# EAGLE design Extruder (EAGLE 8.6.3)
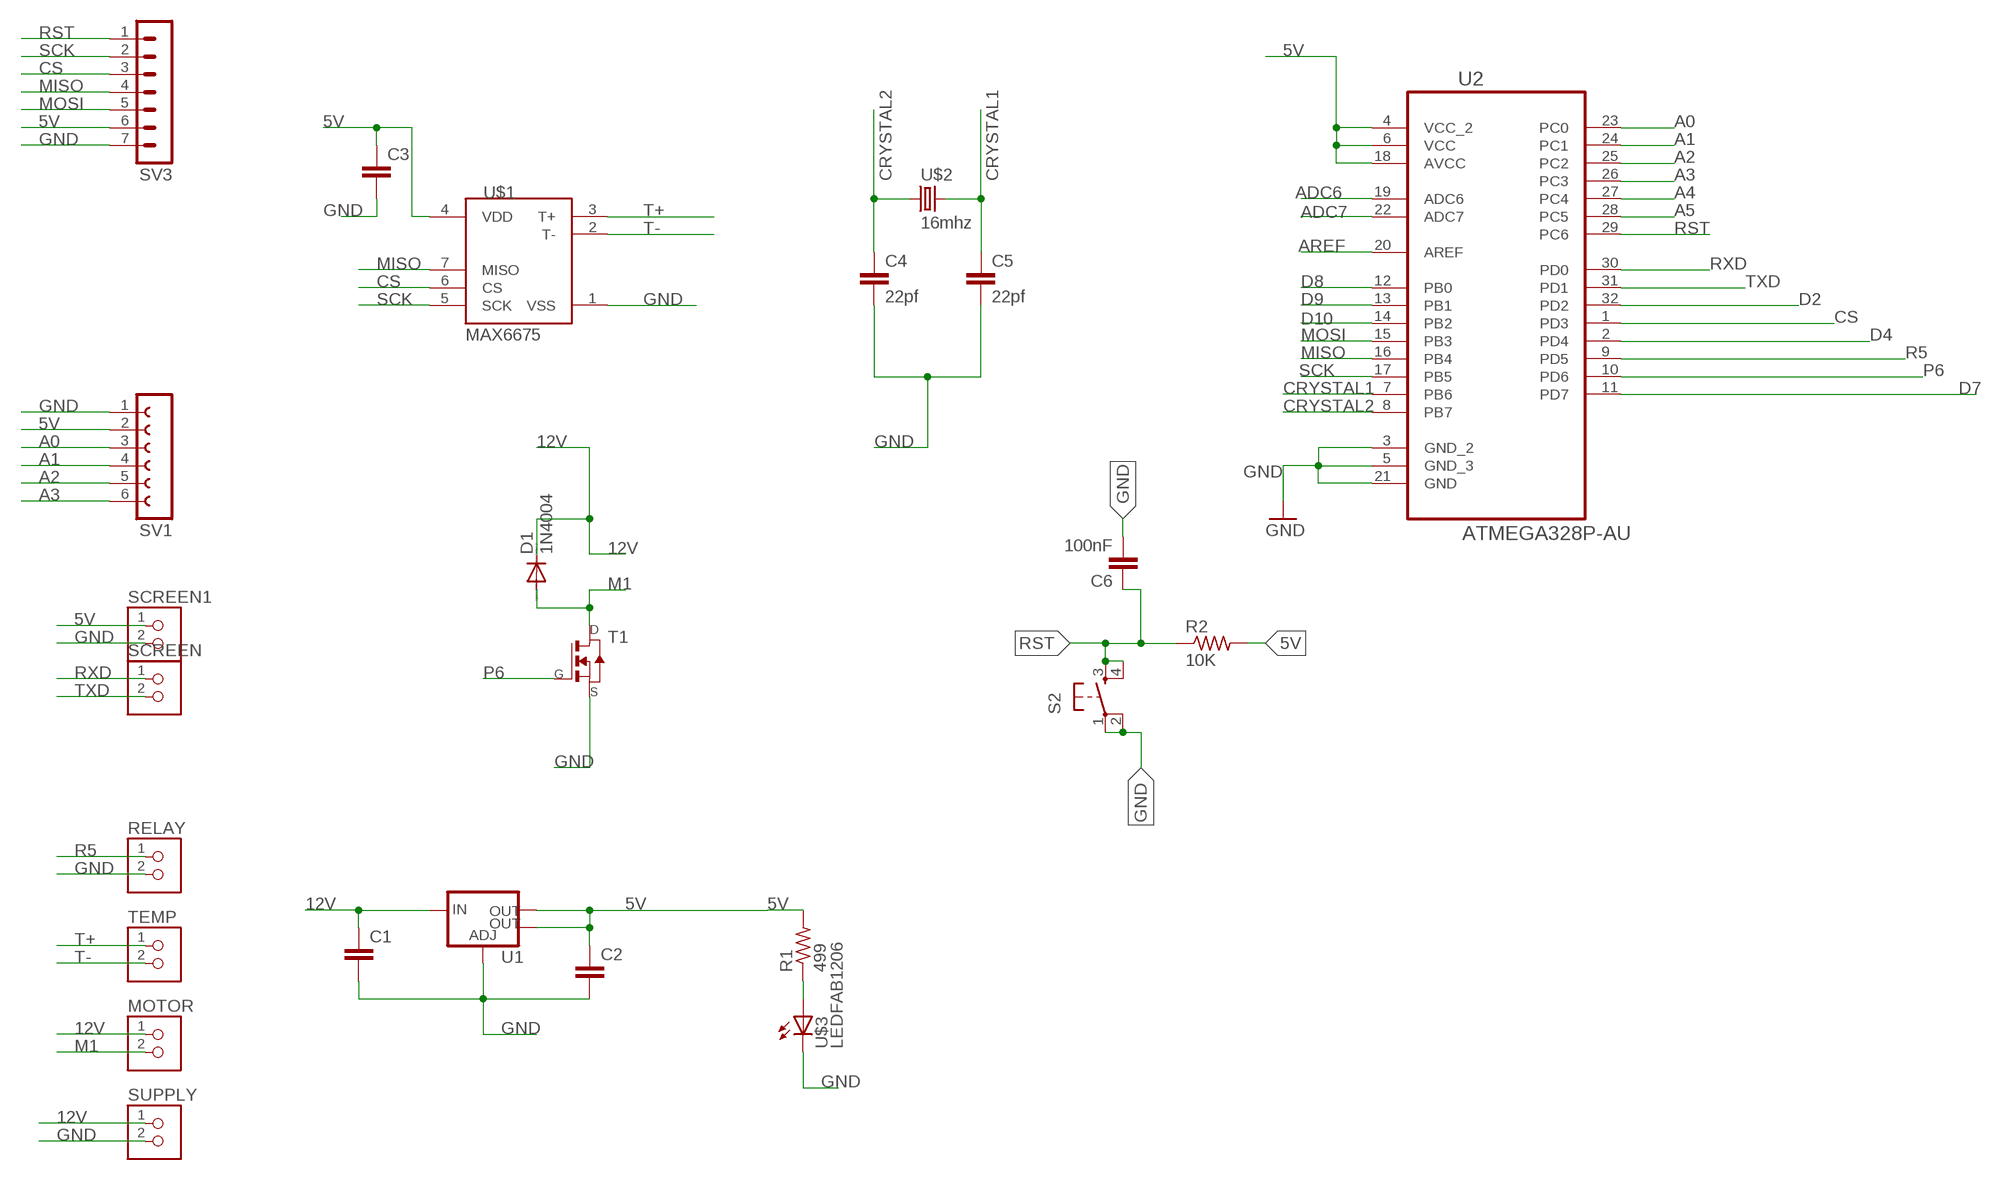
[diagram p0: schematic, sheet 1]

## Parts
C1  C-EUC1206  [C1206]
C2  C-EUC1206  [C1206]
C3  C-EUC1206  [C1206]
C4  22pf  C-EUC1206  [C1206]
C5  22pf  C-EUC1206  [C1206]
C6  100nF  CAP1206  [1206]
D1  1N4004  [DO41-10]
MOTOR  TERM-1X02-FABLAB  [ED555DS-2DS]
R1  499  RES-US1206FAB  [R1206FAB]
R2  10K  RES-US1206FAB  [R1206FAB]
RELAY  TERM-1X02-FABLAB  [ED555DS-2DS]
S2  6MM_SWITCH6MM_SWITCH  [6MM_SWITCH]
SCREEN  TERM-1X02-FABLAB  [ED555DS-2DS]
SCREEN1  TERM-1X02-FABLAB  [ED555DS-2DS]
SUPPLY  TERM-1X02-FABLAB  [ED555DS-2DS]
SV1  FE06-1  [FE06]
SV3  MA07-1  [MA07-1]
T1  NMOSFETTO252  [TO252]
TEMP  TERM-1X02-FABLAB  [ED555DS-2DS]
U1  V_REG_LM1117SOT223  [SOT223]
U2  ATMEGA328P-AU  [QFP80P900X900X120-32N]
U$1  MAX6675  [SO08-MAX6675]
U$2  16mhz  CRYSTAL  [2-SMD-5X3MM]
U$3  LEDFAB1206  [LED1206FAB]

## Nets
5V: C2.1 C3.1 R1.2 R2.2 SCREEN1.1 SV1.2 SV3.6 U1.2(OUT) U1.4(OUT) U2.4(VCC_2) U2.6(VCC) U2.18(AVCC) U$1.4(VDD)
12V: C1.1 D1.C MOTOR.1 SUPPLY.1 U1.3(IN)
A0: SV1.3 U2.23(PC0)
A1: SV1.4 U2.24(PC1)
A2: SV1.5 U2.25(PC2)
A3: SV1.6 U2.26(PC3)
A4: U2.27(PC4)
A5: U2.28(PC5)
ADC6: U2.19(ADC6)
ADC7: U2.22(ADC7)
AREF: U2.20(AREF)
CRYSTAL1: C5.1 U2.7(PB6) U$2.P$2
CRYSTAL2: C4.1 U2.8(PB7) U$2.P$1
CS: SV3.3 U2.1(PD3) U$1.6(CS)
D2: U2.32(PD2)
D4: U2.2(PD4)
D7: U2.11(PD7)
D8: U2.12(PB0)
D9: U2.13(PB1)
D10: U2.14(PB2)
GND: C1.2 C2.2 C3.2 C4.2 C5.2 C6.2 RELAY.2 S2.1(P) S2.2(P1) SCREEN1.2 SUPPLY.2 SV1.1 SV3.7 T1.2(S) U1.1(ADJ) U2.3(GND_2) U2.5(GND_3) U2.21(GND) U$1.1(VSS) U$3.2(C)
M1: D1.A MOTOR.2 T1.3(D)
MISO: SV3.4 U2.16(PB4) U$1.7(MISO)
MOSI: SV3.5 U2.15(PB3)
N$1: R1.1 U$3.1(A)
P6: T1.1(G) U2.10(PD6)
R5: RELAY.1 U2.9(PD5)
RST: C6.1 R2.1 S2.3(S) S2.4(S1) SV3.1 U2.29(PC6)
RXD: SCREEN.1 U2.30(PD0)
SCK: SV3.2 U2.17(PB5) U$1.5(SCK)
T+: TEMP.1 U$1.3(T+)
T-: TEMP.2 U$1.2(T-)
TXD: SCREEN.2 U2.31(PD1)

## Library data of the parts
C1-C5 = rcl:C-EU: CAPACITOR, European symbol; SPICEPREFIX: C
C6 = 01_SparkFun:CAP: Capacitor
D1 = diode:1N4004: DIODE
MOTOR RELAY SCREEN SCREEN1 SUPPLY TEMP = fab:TERM-1X02: 3.5mm terminal block, 2 positions ED555-2DS as found in the fablab inventory.
R1 R2 = fab:RES-US: Resistor (US Symbol)
S2 = fab:6MM_SWITCH: OMRON SWITCH
SV1 = con-lsta:FE06-1: FEMALE HEADER; OC_FARNELL: unknown; OC_NEWARK: unknown
SV3 = con-lstb:MA07-1: PIN HEADER; OC_FARNELL: unknown; OC_NEWARK: unknown
T1 = fab:NMOSFET: MOS FET
U1 = fab:V_REG_LM1117: Voltage Regulator LM1117 Standard adjustable voltage regulator but in SMD form. Spark Fun Electronics SKU : COM-00595; PROD_ID: VREG-08170
U2 = ATMEGA328P-AU:ATMEGA328P-AU: 8-bit Microcontroller with In-System Programmable Flash; AVAILABILITY: Good; DESCRIPTION: ATmega Series 20 MHz 32 KB Flash 2 KB SRAM 8-Bit Microcontroller - TQFP-32; MF: Microchip; MP: ATMEGA328P-AU; PACKAGE: TQFP-32 Atmel; PRICE: 2.09 USD
U$1 = max6675:MAX6675
U$2 = fab:CRYSTAL
U$3 = fab:LED: LED

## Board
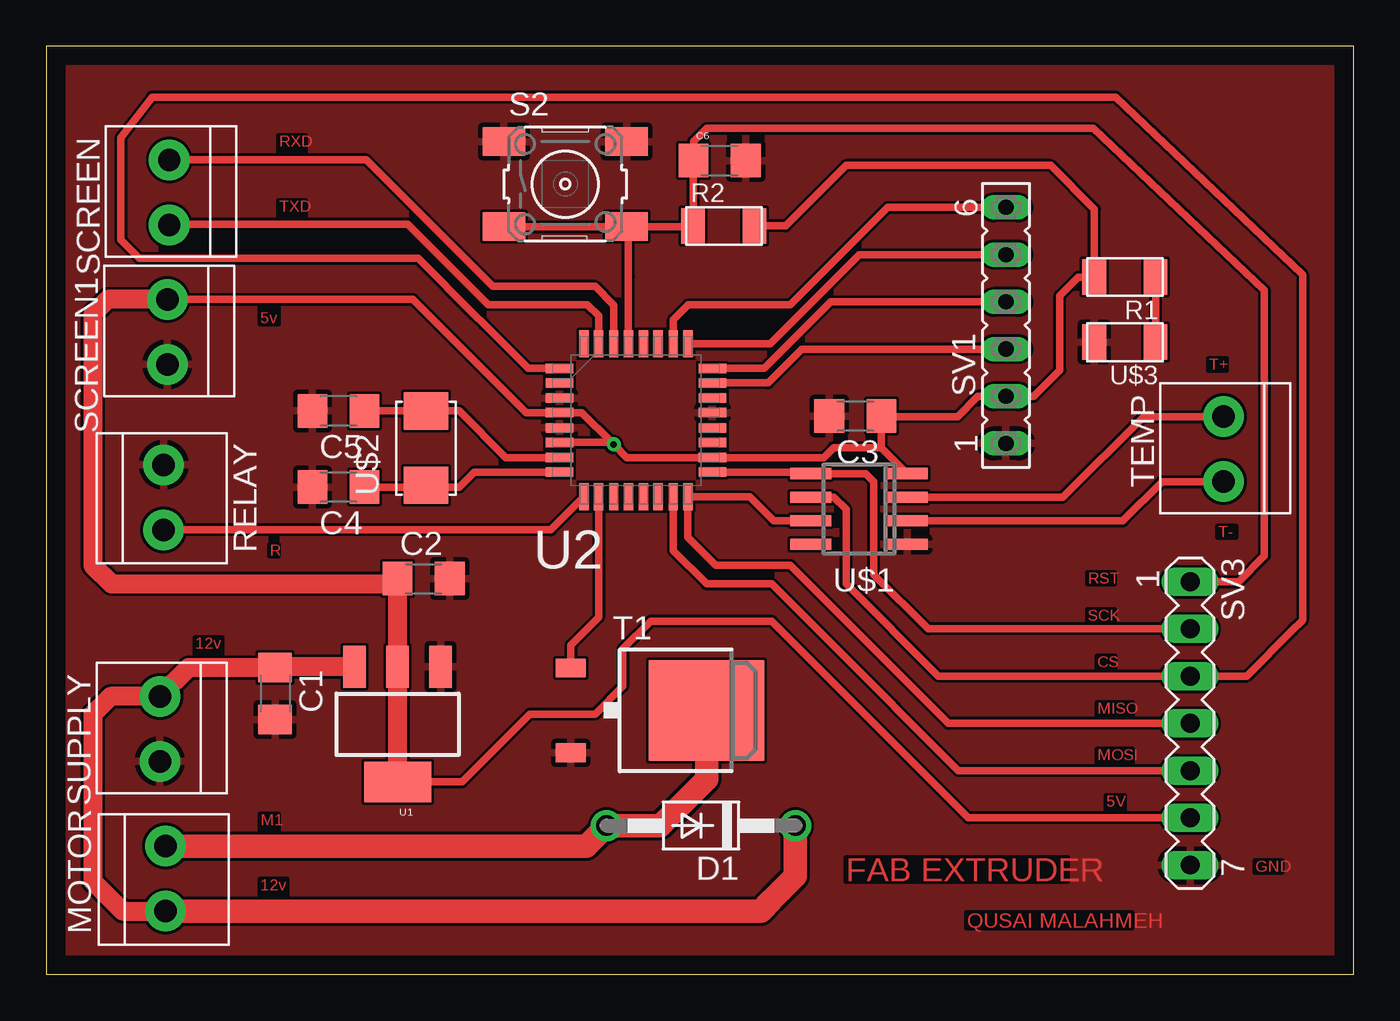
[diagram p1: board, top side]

Size 70.29 x 49.9 mm. Coordinates in mm from the lower left corner, seen from the top.
Outline: 0,0 70.29,0 70.29,49.9 0,49.9 0,0
Copper layers (1*16): Top 0.035mm / dielectric 1.5mm / Bottom 0.035mm
Design rules "default": minimum track width 6mil, minimum drill 0.35mm, track to track 6mil, track to pad 6mil, pad to pad 6mil, via to via 6mil, smd to smd 6mil, copper to edge 40mil, drill to drill 6mil, minimum pad ring 10mil, minimum via ring 8mil, stop-mask expansion 4mil, vias tented up to drill 0mil, thermal gap 10mil

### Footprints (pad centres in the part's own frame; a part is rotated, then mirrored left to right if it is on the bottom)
C1206 = smd 1.6 x 1.8: 1 -1.4,0; 2 1.4,0
1206 = smd 1.6 x 1.8: 1 -1.4,0; 2 1.4,0
DO41-10 = drill 1.118: A 5.08,0; C -5.08,0
ED555DS-2DS = drill 1.2 pad 2.184: 1 1.8,0; 2 -1.7,0
R1206FAB = smd 1.27 x 1.905: 1 -1.651,0; 2 1.651,0
6MM_SWITCH = smd 2.286 x 1.524: 1 -3.302,2.286; 2 3.302,2.286; 3 -3.302,-2.286; 4 3.302,-2.286
FE06 = drill 0.813 long: 1 -6.35,0; 2 -3.81,0; 3 -1.27,0; 4 1.27,0; 5 3.81,0; 6 6.35,0
MA07-1 = drill 1.016 long: 1 -7.62,0; 2 -5.08,0; 3 -2.54,0; 4 0,0; 5 2.54,0; 6 5.08,0; 7 7.62,0
TO252 = smd 1 x 1.6: 1 -2.28,-4.8; 2 2.28,-4.8 | smd 5.4 x 6.2: 3 0,2.5
SOT223 = smd 1.219 x 2.235: 1 -2.311,-3.099; 2 0,-3.099; 3 2.311,-3.099 | smd 3.6 x 2.2: 4 0,3.099
QFP80P900X900X120-32N = smd 1.473 x 0.508: 1 -4.115,2.794; 2 -4.115,2.007; 3 -4.115,1.194; 4 -4.115,0.406; 5 -4.115,-0.406; 6 -4.115,-1.194; 7 -4.115,-2.007; 8 -4.115,-2.794; 17 4.115,-2.794; 18 4.115,-2.007; 19 4.115,-1.194; 20 4.115,-0.406; 21 4.115,0.406; 22 4.115,1.194; 23 4.115,2.007; 24 4.115,2.794 | smd 0.508 x 1.473: 9 -2.794,-4.115; 10 -2.007,-4.115; 11 -1.194,-4.115; 12 -0.406,-4.115; 13 0.406,-4.115; 14 1.194,-4.115; 15 2.007,-4.115; 16 2.794,-4.115; 25 2.794,4.115; 26 2.007,4.115; 27 1.194,4.115; 28 0.406,4.115; 29 -0.406,4.115; 30 -1.194,4.115; 31 -2.007,4.115; 32 -2.794,4.115
SO08-MAX6675 = smd 0.6 x 2.2: 1 -1.905,-2.6; 2 -0.635,-2.6; 3 0.635,-2.6; 4 1.905,-2.6; 5 1.905,2.6; 6 0.635,2.6; 7 -0.635,2.6; 8 -1.905,2.6
2-SMD-5X3MM = smd 2 x 2.4: P$1 -2,0; P$2 2,0
LED1206FAB = smd 1.27 x 1.905: 1 -1.651,0; 2 1.651,0

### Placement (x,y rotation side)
C1  12.3,15.1 270 top
C2  20.28,21.28 0 top
C3  43.5,30.02 180 top
C4  15.7,26.2 180 top
C5  15.7,30.3 180 top
C6  36.2,43.77 0 top
D1  35.2,8 180 top
MOTOR  6.4,5.2 270 top
R1  58,37.5 180 top
R2  36.43,40.25 0 top
RELAY  6.3,25.7 270 top
S2  27.9,42.5 0 top
SCREEN  6.6,42 90 top
SCREEN1  6.5,34.5 90 top
SUPPLY  6.1,13.15 90 top
SV1  51.6,34.9 90 top
SV3  61.5,13.5 270 top
T1  33,14.2 270 top
TEMP  63.3,28.2 90 top
U1  18.88,13.45 180 top
U2  31.7,29.8 0 top
U$1  43.7,25.03 90 top
U$2  20.4,28.3 90 top
U$3  58,34 180 top

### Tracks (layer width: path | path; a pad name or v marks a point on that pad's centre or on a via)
5V  (via drill 0.35)
  Top 0.406: U2.6 30.39,28.61 | 30.39,28.61 28.79,30.21 U2.4 25.79,30.21 19.7,36.3 SCREEN1.1 | 30.39,28.61 v30.5,28.5 31.21,27.79 U2.18 41.79,27.79 42.33,28.33 44.9,28.33 | 37.96,39.87 R2.2 39.75,40.25 43,43.5 54,43.5 56.35,41.15 R1.2 55.5,37.5 54.5,36.5 54.5,32.5 53.09,31.09 SV1.2 50.09,31.09 49,30 44.92,30 C3.1 44.9,28.33 | U1.4 22.35,10.35 26,14 29.5,14 31,15.5 31,17.5 32.5,19 39,19 49.58,8.42 SV3.6 | U$1.4 44.9,28.33
  Top 1.016: U1.4 U1.2 C2.1 18.6,21 3.5,21 2.5,22 2.5,35.5 3.3,36.3 SCREEN1.1
12V
  Top 1.016: U1.3 12.35,16.55 | C1.1 7.65,16.5 SUPPLY.1 3.45,14.95 2.5,14 2.5,5 4.1,3.4 MOTOR.1
  Top 1.27: C1.1 12.35,16.55 | MOTOR.1 38.4,3.4 39,4 39.5,4.5 40.28,5.28 D1.C
A0
  Top 0.406: SV1.3 40.63,33.63 38.81,31.81 U2.23
A1
  Top 0.406: U2.24 38.59,32.59 42.17,36.17 SV1.4
A2
  Top 0.406: U2.25 38.91,33.91 43.71,38.71 SV1.5
A3
  Top 0.406: U2.26 33.71,35.21 34.5,36 40,36 45.25,41.25 SV1.6
CRYSTAL1
  Top 0.406: C5.1 20,30.3 U$2.P$2 22.2,30.3 24.71,27.79 U2.7
CRYSTAL2
  Top 0.406: C4.1 19.5,26.2 20.3,26.2 | 20.3,26.2 U$2.P$1 | U2.8 23.01,27.01 22.2,26.2 20.3,26.2
CS
  Top 0.406: U$1.6 42.34,25.66 43,25 43,21 47.96,16.04 SV3.3 64.54,16.04 67,18.5 67.5,19 67.56,19.06 67.56,37.62 57.5,47.18 5.68,47.18 4,45 4,39.5 5,38.5 19.98,38.5 23.02,35.46 23.54,34.96 25.91,32.59 U2.1
GND
  pour Top: 0,-0.5 70.31,-0.5 70.31,51.23 0,51.23
M1
  Top 1.27: MOTOR.2 29.02,6.9 D1.A 33,8 35.5,10.5 T1.3
MISO
  Top 0.406: U$1.7 39.11,24.39 37.81,25.68 U2.16 34.49,23.51 36,22 40,22 45,17 45.09,16.91 48.5,13.5 SV3.4
MOSI
  Top 0.406: U2.15 33.71,22.79 35.5,21 39,21 45.5,14.5 45.63,14.37 49.04,10.96 SV3.5
N$1
  Top 0.406: U$3.1 R1.1
P6
  Top 0.406: U2.10 29.69,19.19 28.2,17.7 T1.1
R5
  Top 0.406: U2.9 27.12,23.9 RELAY.1
RST
  Top 0.406: U2.29 31.29,37.5 | 31.29,37.51 31.29,37.5 | S2.3 S2.4 | 31.29,37.5 31.29,40.12 S2.4 | SV3.1 64.12,21.12 65.5,22.5 65.5,36.79 56.29,45.5 35.5,45.5 34.8,44.8 C6.1 34.78,43.74 R2.1 34.74,40.21 S2.4
RXD
  Top 0.406: U2.30 30.51,35.99 29.5,37 24,37 17.2,43.8 SCREEN.1
SCK
  Top 0.406: U2.17 41.03,27.01 U$1.5 44.07,26.93 44.5,26.5 44.5,21.5 47.42,18.58 SV3.2
T+
  Top 0.406: U$1.3 54.66,25.66 59,30 TEMP.1
T-
  Top 0.406: U$1.2 57.89,24.39 60,26.5 TEMP.2
TXD
  Top 0.406: U2.31 29.69,35.41 29.08,36.02 23.75,36.02 19.43,40.34 6.64,40.34 SCREEN.2

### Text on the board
Top: RXD | TXD | 5v | T+ | T- | R | RST | SCK | 12v | CS | MISO | MOSI | 5V | M1 | GND | FAB EXTRUDER | 12v | QUSAI MALAHMEH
